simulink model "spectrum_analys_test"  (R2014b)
settings: Solver=ode45  StartTime=0.0  StopTime=10  RelTol=1e-3
undefined symbols (not defined in the file or in its folder): get
libraries: dspstat3 x3, simulink x1, dspsnks4 x1

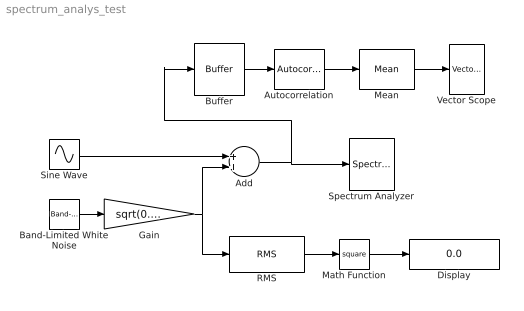
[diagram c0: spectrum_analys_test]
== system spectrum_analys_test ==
  Add : Sum
  Autocorrelation : dspstat3/Autocorrelation  AllPositiveLags=on  maxlag=1  bias=Biased  domain=Time  outputDataTypeStr=Inherit: Same as accumulator  outputLastDataTypeStr=Inherit: Same as accumulator  outputMin=[]  outputMax=[]  roundingMode=Floor  overflowMode=off
  Band-Limited White Noise : simulink/Sources/Band-Limited White Noise  Cov=1/5000  Ts=1/5000  seed=[23341]
  Buffer : Buffer  N=1024  TreatMby1Signals=One channel
  Display : Display
  Gain : Gain  Gain=sqrt(0.01)
  Math Function : Math  Operator=square
  Mean : dspstat3/Mean  run=on  reset_popup=None  directionMode=Each column  dimension=1  treatSBRowAsCol=on  roiEnable=off  roiType=Rectangles  roiPortion=Entire ROI  roiOutput=Individual statistics for each ROI  roiFlag=off  outputDataTypeStr=Inherit: Same as accumulator  outputLastDataTypeStr=Inherit: Same as accumulator  outputMin=[]  outputMax=[]  roundingMode=Floor  overflowMode=off
  RMS : dspstat3/RMS  run=on  reset_popup=None  directionMode=Each column  dimension=1  treatSBRowAsCol=on
  Sine Wave : Sin  Frequency=2*pi*100  SampleTime=1/5000
  Spectrum Analyzer : SpectrumAnalyzer
  Vector Scope : dspsnks4/Vector Scope  ScopeProperties=on  Domain=Time  HorizSpan=1  DisplayProperties=off  AxisGrid=on  Memory=off  FrameNumber=on  AxisLegend=off  AxisZoom=off  OpenScopeAtSimStart=on  OpenScopeImmediately=off  FigPos=get(0,'defaultfigureposition')  AxisProperties=off  XUnits=Hertz  XRange=[0...Fs/2]  InheritXIncr=on  XIncr=1  XLabel=Time  XLimit=Auto  XMin=0  XMax=1  XStart=0  YUnits=dB  YLabel=Amplitude  LineProperties=off  XAxisParamsVer=6.9
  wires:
  Band-Limited White Noise/1 -> Gain/1
  Sine Wave/1 -> Add/1
  Gain/1 -> RMS/1, Add/2
  Add/1 -> Buffer/1, Spectrum Analyzer/1
  RMS/1 -> Math Function/1
  Math Function/1 -> Display/1
  Buffer/1 -> Autocorrelation/1
  Autocorrelation/1 -> Mean/1
  Mean/1 -> Vector Scope/1
